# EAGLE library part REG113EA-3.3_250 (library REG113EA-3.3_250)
400mA, Low-Noise, Low-Dropout Regulator Source: Datasheet
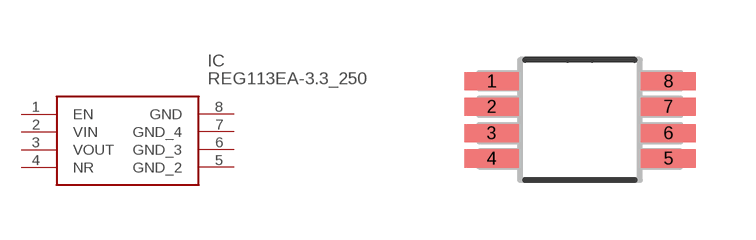
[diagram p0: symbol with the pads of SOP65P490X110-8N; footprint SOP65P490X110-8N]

Designator prefix IC

## REG113EA-3.3_250 (Description: 400mA, Low-Noise, Low-Dropout Regulator; Height: mm; Manufacturer_Name: Texas Instruments; Manufacturer_Part_Number: REG113EA-3.3/250; Mouser_Part_Number: 595-REG113EA-3.3/250; Mouser_Price-Stock: https://www.mouser.co.uk/ProductDetail/Texas-Instruments/REG113EA-33-250?qs=sSOk4GDDv7xPko1XdFasfg%3D%3D)  [SOP65P490X110-8N]
1  EN
2  VIN
3  VOUT
4  NR
5  GND_2
6  GND_3
7  GND_4
8  GND

## Footprint SOP65P490X110-8N (pad centres in mm)
SOP65P490X110-8N
smd 1.372 x 0.457: 1 -2.21,0.965; 2 -2.21,0.33; 3 -2.21,-0.33; 4 -2.21,-0.965; 5 2.21,-0.965; 6 2.21,-0.33; 7 2.21,0.33; 8 2.21,0.965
